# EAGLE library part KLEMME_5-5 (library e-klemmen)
Klemme 5 5
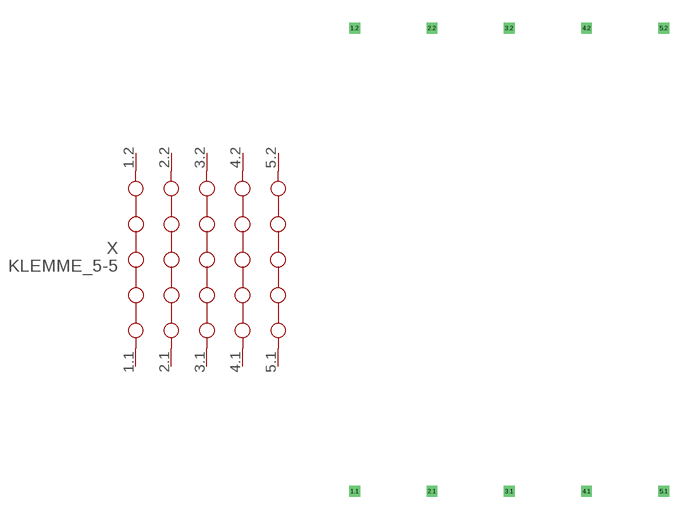
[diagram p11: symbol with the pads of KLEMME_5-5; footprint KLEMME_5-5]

Designator prefix X

## KLEMME_5-5  [KLEMME_5-5]
1.1  1.1  pas
1.2  1.2  pas
2.1  2.1  pas
2.2  2.2  pas
3.1  3.1  pas
3.2  3.2  pas
4.1  4.1  pas
4.2  4.2  pas
5.1  5.1  pas
5.2  5.2  pas

## Footprint KLEMME_5-5 (pad centres in mm)
Dummy
drill 0.2 pad 0.6 square: 1.1 0,-15.24; 1.2 0,15.24; 2.1 5.08,-15.24; 2.2 5.08,15.24; 3.1 10.16,-15.24; 3.2 10.16,15.24; 4.1 15.24,-15.24; 4.2 15.24,15.24; 5.1 20.32,-15.24; 5.2 20.32,15.24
